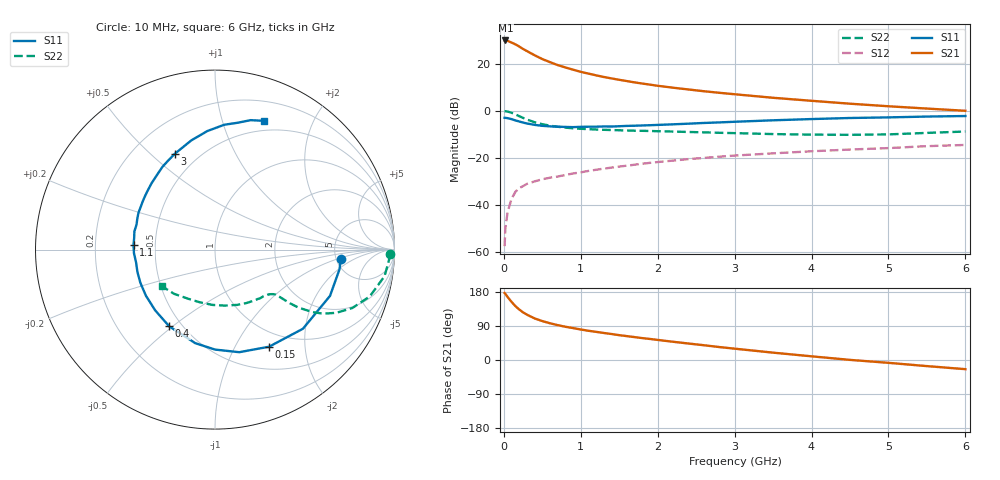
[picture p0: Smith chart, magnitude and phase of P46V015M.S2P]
! SIEMENS Small Signal Semiconductors
! BFP182
! Si NPN RF Bipolar Junction Transistor in SOT143
! VCE = 6 V  IC = 15 mA
! Common Emitter S-Parameters:  March  1996
# GHz  S  MA  R  50
!  f  S11  S21  S12  S22
! GHz  MAG  ANG  MAG  ANG  MAG  ANG  MAG  ANG
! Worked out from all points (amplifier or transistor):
!   36 points, 10 MHz to 6 GHz, reference 50 ohm
!   highest |S21| = 29.9 dB at 20 MHz (marker M1)
!   |S21| within 3 dB of that: start of sweep to 220.2 MHz
!   unconditionally stable (mu >= 1): 998.5 MHz to 5.43 GHz
!   at 250 MHz: K = 0.39, MSG = 29.2 dB, |S12| = -32.1 dB
!   at 1.4 GHz: K = 1.10, MAG = 17.0 dB, |S12| = -24.3 dB
!   at 6 GHz: K = 0.95, MSG = 7.3 dB, |S12| = -14.6 dB
!   S11 on the Smith chart (normalised r, x): 10 MHz: 5.49, -1.15; 150 MHz: 0.79, -1.39; 400 MHz: 0.43, -0.49; 1.1 GHz: 0.38, +0.02; 3 GHz: 0.37, +0.60; 6 GHz: 0.39, +1.38
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0.01  0.7033 -4.3  31.08 176.7  0.0013 86.5  0.9737 -1.5
0.02  0.7023 -9.0  31.22 174.4  0.0032 77.6  0.9712 -3.5
0.05  0.6908 -21.9  30.58 166.0  0.007 81.5  0.9563 -8.9
0.1  0.6591 -42.0  28.19 153.5  0.0132 71.0  0.9012 -16.8
0.15  0.6192 -60.9  25.83 142.2  0.0186 63.0  0.832 -23.0
0.2  0.5874 -76.7  23.19 133.2  0.0224 58.7  0.7626 -27.5
0.25  0.557 -90.0  20.59 125.7  0.0247 55.2  0.7015 -30.6
0.3  0.5328 -101.9  18.54 119.7  0.0276 52.4  0.6465 -32.6
0.4  0.4979 -120.8  15.1 109.7  0.0311 49.6  0.5666 -34.8
0.5  0.475 -134.6  12.53 102.7  0.0346 48.4  0.5144 -35.6
0.6  0.4628 -146.3  10.79 96.9  0.0373 48.5  0.4783 -35.9
0.7  0.4552 -156.0  9.327 92.0  0.0396 48.4  0.4534 -36.1
0.9  0.4454 -170.5  7.447 84.2  0.0459 49.2  0.4205 -36.6
1.1  0.4547 176.8  6.151 77.1  0.052 49.6  0.4031 -38.0
1.5  0.4654 158.6  4.534 65.5  0.0644 49.2  0.3823 -41.8
1.8  0.4834 146.6  3.775 57.8  0.0741 48.5  0.3716 -45.9
2.2  0.5113 133.8  3.078 48.1  0.0864 46.1  0.3587 -52.3
3  0.5795 112.6  2.234 29.9  0.1104 40.2  0.332 -68.1
3.5  0.6228 102.2  1.878 19.4  0.1231 35.9  0.3169 -79.9
4.5  0.6973 85.8  1.405 0.3  0.1484 27.8  0.3055 -106.3
5.5  0.7481 74.6  1.107 -16.1  0.1753 20.2  0.3358 -132.8
6  0.7679 69.1  0.993 -24.2  0.186 15.4  0.3592 -145.4
